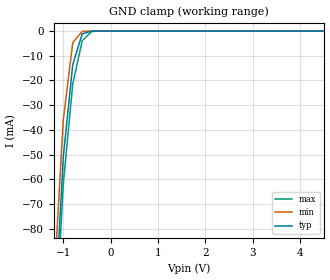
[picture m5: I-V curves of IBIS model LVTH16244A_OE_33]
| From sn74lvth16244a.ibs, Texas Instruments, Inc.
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|  Model LVTH16244A Input_OE_33
[Model]   LVTH16244A_OE_33
Model_type  Input
Polarity   Inverting
Vinl = 0.8V
Vinh = 2.0V
| variable   typ   min   max
C_comp   4pf   NA   NA
[Temperature Range]   40   -25   100
| Ambient temperature   25   -40   85
[Voltage range]   3.3   3.0   3.6
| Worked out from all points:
|   GND clamp passes 1 mA (typ) near -0.58 V on its own axis
[GND Clamp]
|   Voltage   I(typ)   I(min)   I(max)
-5V       -2.039A    -2.406A    -1.824A
-1.2V     -122.1mA   -103.4mA   -132.9mA
-1V       -50.9mA    -35.99mA   -61.95mA
-800mV    -13.52mA   -4.664mA   -21.4mA
-600mV    -1.087mA   -123.6uA   -3.906mA
-400mV    -5.587uA   -278.4nA   -154.6uA
-200mV    -4.859nA   -103.4nA   -482.3nA
5V        103.8pA    224nA      360.8pA
